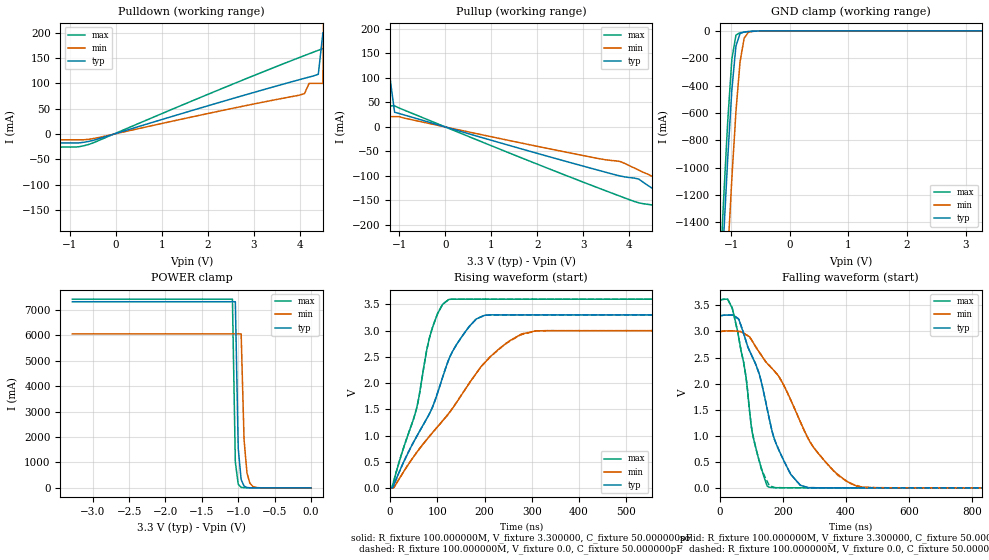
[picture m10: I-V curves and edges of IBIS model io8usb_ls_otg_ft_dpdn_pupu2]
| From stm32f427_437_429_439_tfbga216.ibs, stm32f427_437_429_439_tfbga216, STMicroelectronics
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|   Model io8usb_ls_otg_ft_dpdn_pupu2
[Model]  io8usb_ls_otg_ft_dpdn_pupu2
Model_type I/O
Polarity   Non-Inverting
Enable   Active-Low
Vinl =   0.990000V
Vinh =   2.310000V
Vmeas =  1.650000V
Cref =   50.000000pF
Rref =   100.000000M
Vref =   0.0V
C_comp   8.255900pF   7.991100pF   8.650600pF
[Temperature Range]   25.000000   0.125000k   -40.000000
[Pullup Reference]   3.300000V   3.000000V   3.600000V
[Pulldown Reference]   0.0V   0.0V   0.0V
[POWER Clamp Reference]   3.300000V   3.000000V   3.600000V
[GND Clamp Reference]   0.0V   0.0V   0.0V
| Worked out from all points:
|   slope of the pulldown table from 0 to 0.495 V, typ, clamps not added: 36.1 ohm
|   slope of the pullup table from 0 to 0.495 V, typ, clamps not added: 36.5 ohm
|   GND clamp passes 1 mA (typ) near -0.52 V on its own axis
|   POWER clamp passes 1 mA (typ) near -0.80 V on its own axis
|   rising waveform, R_fixture 100.000000M, V_fixture 3.300000, C_fixture 50.000000pF: 20-80 % time 96.9ns typ, 151ns min, 56.9ns max; typ from 0.008 V to 3.3 V
|   rising waveform, R_fixture 100.000000M, V_fixture 0.0, C_fixture 50.000000pF: 20-80 % time 96.9ns typ, 151ns min, 56.9ns max; typ from 0.008 V to 3.3 V
|   falling waveform, R_fixture 100.000000M, V_fixture 3.300000, C_fixture 50.000000pF: 20-80 % time 98.6ns typ, 172ns min, 55.9ns max; typ from 3.3 V to 0.008 V
|   falling waveform, R_fixture 100.000000M, V_fixture 0.0, C_fixture 50.000000pF: 20-80 % time 98.6ns typ, 172ns min, 55.9ns max; typ from 3.3 V to 0.008 V
[Pulldown]
|Voltage   I(typ)   I(min)   I(max)
-3.3V     -182mA     -11.2mA    -25.53mA
-3.2V     -17.29mA   -11.2mA    -25.53mA
-600mV    -14.61mA   -10.33mA   -20.77mA
4V        107.6mA    77mA       151.4mA
4.1V      110mA      80mA       154.9mA
4.2V      112.5mA    100mA      158.4mA
4.4V      118mA      100mA      165.2mA
4.5V      200mA      100mA      168.6mA
4.6V      200mA      1A         172mA
4.7V      200mA      1A         176mA
4.8V      1A         1A         200mA
6.6V      1A         1A         1A
[Pullup]
|Voltage   I(typ)   I(min)   I(max)
-3.3V     1A         1A         1A
-1.9V     1A         1A         1A
-1.8V     100mA      1A         1A
-1.7V     100mA      1A         100mA
-1.6V     100mA      1A         100mA
-1.5V     100mA      21mA       100mA
-1.3V     100mA      21mA       100mA
-1.2V     100mA      21mA       43mA
-1.1V     30mA       21mA       43mA
4.2V      -106.4mA   -88.1mA    -154.8mA
5V        -155.6mA   -124mA     -201.7mA
6.6V      -222mA     -161mA     -319mA
[GND_clamp]
|Voltage   I(typ)   I(min)   I(max)
-3.3V     -9.433A    -9.435A    -9.911A
-1.2V     -2.116A    -2.846A    -1.847A
-1.13V    -1.505A    -2.23A     -1.23A
-1.06V    -930.4mA   -1.637A    -658.9mA
-990mV    -432.7mA   -1.08A     -207.3mA
-920mV    -110.5mA   -590.3mA   -31.59mA
-850mV    -19.84mA   -226.8mA   -13.66mA
-780mV    -8.32mA    -54.05mA   -9.516mA
-710mV    -5.29mA    -11.97mA   -6.271mA
-640mV    -3.236mA   -4.296mA   -3.584mA
3.28V     0A         0A         0A
[POWER_clamp]
|Voltage   I(typ)   I(min)   I(max)
-3.28V    7.329A     6.064A     7.431A
-1.08V    7.329A     6.064A     7.431A
-1.04V    7.329A     6.064A     1.016A
-1V       1.545A     6.064A     139.4mA
-960mV    326.1mA    6.064A     19.66mA
-920mV    69.13mA    1.89A      3.273mA
-880mV    14.93mA    589.3mA    2.081mA
-840mV    3.481mA    183.9mA    2.081mA
-800mV    1.046mA    57.51mA    2.081mA
-720mV    377.9uA    5.818mA    2.081mA
0V        102.7nA    83.74nA    311.9nA
[Ramp]
| variable   typ   min   max
dV/dt_r  1.45122/0.11073u   1.20359/0.19784u   1.71494/65.08987n
dV/dt_f  1.45552/95.08162n   1.20641/0.16624u   1.71727/55.24844n
R_load = 100.000000
[Rising Waveform]
R_fixture= 100.000000M
V_fixture= 3.300000
V_fixture_min= 3.000000
V_fixture_max= 3.600000
C_fixture= 50.000000pF
|time   V(typ)   V(min)   V(max)
0s        7.865mV    8.028mV    8.988mV
4.004ns   7.236mV    8.015mV    11.18mV
54.72ns   958.2mV    659.4mV    1.468V
88.09ns   1.506V     1.039V     3.007V
110.8ns   2.098V     1.277V     3.492V
125.5ns   2.475V     1.438V     3.596V
182.8ns   3.224V     2.192V     3.6V
252.3ns   3.3V       2.802V     3.6V
308.3ns   3.3V       2.995V     3.6V
1.333us   3.3V       3V         3.6V
[Rising Waveform]
R_fixture= 100.000000M
V_fixture= 0.0
V_fixture_min= 0.0
V_fixture_max= 0.0
C_fixture= 50.000000pF
|time   V(typ)   V(min)   V(max)
0s        7.864mV    8.027mV    8.987mV
54.72ns   958.1mV    659.4mV    1.468V
77.41ns   1.32V      922.9mV    2.617V
89.42ns   1.534V     1.053V     3.045V
110.8ns   2.098V     1.278V     3.495V
125.5ns   2.475V     1.438V     3.597V
182.8ns   3.224V     2.192V     3.6V
244.2ns   3.3V       2.749V     3.6V
308.3ns   3.3V       2.993V     3.6V
1.333us   3.3V       3V         3.6V
[Falling Waveform]
R_fixture= 100.000000M
V_fixture= 3.300000
V_fixture_min= 3.000000
V_fixture_max= 3.600000
C_fixture= 50.000000pF
|time   V(typ)   V(min)   V(max)
0s        3.3V       3V         3.6V
41.37ns   3.312V     3.01V      3.418V
82.75ns   2.834V     2.94V      2.164V
104.1ns   2.508V     2.807V     1.052V
153.5ns   1.437V     2.371V     29.8mV
190.9ns   688.5mV    2.103V     9.641mV
254.9ns   61.6mV     1.28V      8.999mV
335ns     8.368mV    504.8mV    8.989mV
436.4ns   7.843mV    31.24mV    8.988mV
1.333us   7.854mV    8.027mV    8.988mV
[Falling Waveform]
R_fixture= 100.000000M
V_fixture= 0.0
V_fixture_min= 0.0
V_fixture_max= 0.0
C_fixture= 50.000000pF
|time   V(typ)   V(min)   V(max)
0s        3.3V       3V         3.6V
41.37ns   3.312V     3.01V      3.418V
82.75ns   2.834V     2.94V      2.164V
105.4ns   2.491V     2.794V     1.012V
157.5ns   1.323V     2.346V     49.74mV
198.9ns   584.6mV    2.021V     9.477mV
254.9ns   61.39mV    1.28V      8.968mV
315ns     8.173mV    647.4mV    8.965mV
416.4ns   7.819mV    84.48mV    8.994mV
1.333us   7.853mV    8.028mV    9.013mV
